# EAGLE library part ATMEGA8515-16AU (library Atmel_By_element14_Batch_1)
8-bit Microcontroller
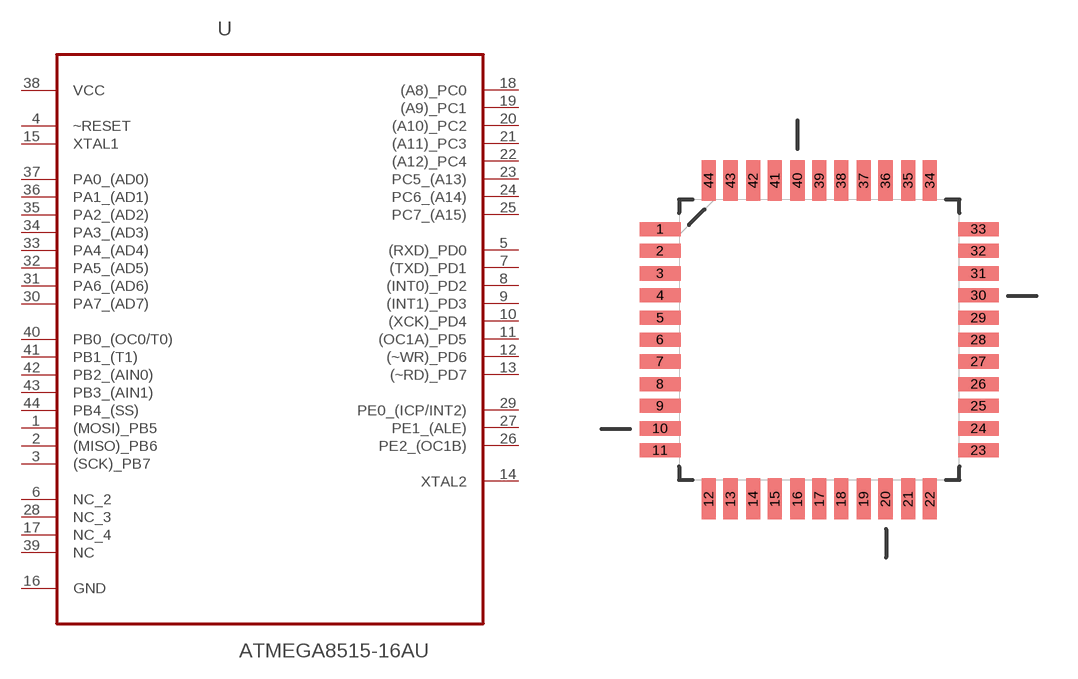
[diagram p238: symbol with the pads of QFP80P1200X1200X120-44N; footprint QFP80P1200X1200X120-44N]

Designator prefix U

## ATMEGA8515-16AU (DESCRIPTION: 8-bit Microcontroller; MPN: ATMEGA8515-16AU; OC_FARNELL: 9171398; OC_NEWARK: 01M6904; PACKAGE: QFP-44; SUPPLIER: Atmel)  [QFP80P1200X1200X120-44N]
1  (MOSI)_PB5
2  (MISO)_PB6
3  (SCK)_PB7
4  ~RESET  in
5  (RXD)_PD0
6  NC_2  nc
7  (TXD)_PD1
8  (INT0)_PD2
9  (INT1)_PD3
10  (XCK)_PD4
11  (OC1A)_PD5
12  (~WR)_PD6
13  (~RD)_PD7
14  XTAL2  out
15  XTAL1  in
16  GND  pas
17  NC_4  nc
18  (A8)_PC0
19  (A9)_PC1
20  (A10)_PC2
21  (A11)_PC3
22  (A12)_PC4
23  PC5_(A13)
24  PC6_(A14)
25  PC7_(A15)
26  PE2_(OC1B)
27  PE1_(ALE)  pwr
28  NC_3  nc
29  PE0_(ICP/INT2)
30  PA7_(AD7)
31  PA6_(AD6)
32  PA5_(AD5)
33  PA4_(AD4)
34  PA3_(AD3)
35  PA2_(AD2)
36  PA1_(AD1)
37  PA0_(AD0)
38  VCC  pwr
39  NC  nc
40  PB0_(OC0/T0)
41  PB1_(T1)
42  PB2_(AIN0)
43  PB3_(AIN1)
44  PB4_(SS)

## Footprint QFP80P1200X1200X120-44N (pad centres in mm)
smd 1.473 x 0.508: 1 -5.74,3.988; 2 -5.74,3.2; 3 -5.74,2.388; 4 -5.74,1.6; 5 -5.74,0.787; 6 -5.74,0; 7 -5.74,-0.787; 8 -5.74,-1.6; 9 -5.74,-2.388; 10 -5.74,-3.2; 11 -5.74,-3.988; 23 5.74,-3.988; 24 5.74,-3.2; 25 5.74,-2.388; 26 5.74,-1.6; 27 5.74,-0.787; 28 5.74,0; 29 5.74,0.787; 30 5.74,1.6; 31 5.74,2.388; 32 5.74,3.2; 33 5.74,3.988
smd 0.508 x 1.473: 12 -3.988,-5.74; 13 -3.2,-5.74; 14 -2.388,-5.74; 15 -1.6,-5.74; 16 -0.787,-5.74; 17 0,-5.74; 18 0.787,-5.74; 19 1.6,-5.74; 20 2.388,-5.74; 21 3.2,-5.74; 22 3.988,-5.74; 34 3.988,5.74; 35 3.2,5.74; 36 2.388,5.74; 37 1.6,5.74; 38 0.787,5.74; 39 0,5.74; 40 -0.787,5.74; 41 -1.6,5.74; 42 -2.388,5.74; 43 -3.2,5.74; 44 -3.988,5.74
